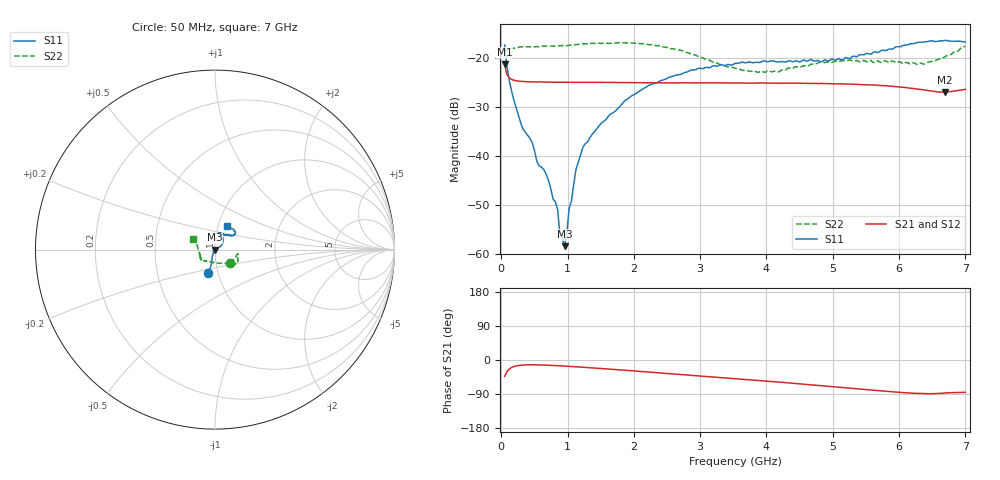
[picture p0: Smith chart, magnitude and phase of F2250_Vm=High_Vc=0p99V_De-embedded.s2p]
! Integrated Device Technology
! Corporate Headquarters
! 6024 Silver Creek Valley Road
! San Jose, CA 95138  USA
! Phone:  1-408-284-8200
! Toll Free:  1-800-223-1366
! Webpage:  http://www.idt.com/
! Timing and RF Division
! 515 Groton Road, Suite 102
! Westford, MA 01886-6024
! Device:  F2250
! Description: Voltage Variable RF Attenuator
! Frequency:  50.0 -  6000.00 MHz
! Package:  3x3 mm Thin QFN Plastic Package: 16 pin
! Ports:  2 RF, 3 DC
!  Pin  1  = GND
!  Pin  2  = NC
!  Pin  3  = RF1  = Port 1
!  Pin  4  = NC
!  Pin  5  = GND
!  Pin  6  = GND
!  Pin  7  = GND
!  Pin  8  = GND
!  Pin  9  = NC
!  Pin 10  = RF2  = Port 2
!  Pin 11  = NC
!  Pin 12  = GND
!  Pin 13  = GND
!  Pin 14  = VCNTRL
!  Pin 15  = VDD
!  Pin 16  = VMODE
! Vcntrl:  0.990 Volts
! Vmode:  +3.300 Volts
! Vdd:  +3.30  Volts
! Current:  1.325 mA
! Data:  The device was measured on a the F2250 evaluation board which has
!  individual transmission lines to the RF pins.  Data was collected
!  using a calibrated network analyzer.  The evaluation board was
!  de-embedded using a TRL calibration technique.
!  The reference plane is the edge of the package pin.
! Misc:  SN 10
!  Action Tracker AT0258
! Date Measured:  2014-11-26
! Date:  2015-10-15  MJV
! Note:
!  Integrated Device Technology supplies this data as a sample of measured
!  data at the package pin for this product.  Your particular data for this
!  product may vary.
!  Data was taken at 25 degrees C.
!  Integrated Device Technology reserves the right to change this data at anytime.
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# GHz S dB R 50
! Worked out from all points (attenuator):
!   201 points, 50 MHz to 7 GHz, reference 50 ohm
!   highest |S21| = -21.20 dB at 50 MHz (marker M1); lowest = -26.9 dB at 6.687 GHz (marker M2)
!   lowest |S11| = -58.4 dB at 953.5 MHz (marker M3), VSWR 1.00, Z = 49.9 - j0.0804 ohm
!   |S11| at or under -10 dB: start of sweep to end of sweep
!   |S22| runs from -22.9 to -16.8 dB; largest |S21 - S12| = 0.00023
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0.05  -17.25 -105.8  -21.20 -43.3  -21.21 -43.3  -19.21 -42.3
0.1195  -24.43 -106.8  -23.97 -24.0  -23.95 -24.0  -18.09 -15.0
0.189  -28.48 -112.3  -24.44 -17.4  -24.43 -17.3  -17.89 -11.6
0.328  -34.45 -120.6  -24.70 -13.3  -24.69 -13.3  -17.59 -10.6
0.467  -37.21 -130.2  -24.79 -12.7  -24.80 -12.7  -17.65 -11.8
0.5365  -41.02 -133.3  -24.81 -12.8  -24.79 -12.8  -17.57 -13.2
0.71025  -44.83 -142.4  -24.84 -13.9  -24.85 -13.9  -17.47 -16.2
0.84925  -50.87 -176.6  -24.86 -15.1  -24.86 -15.1  -17.43 -19.1
0.884  -55.84 175.0  -24.88 -15.4  -24.89 -15.4  -17.39 -20.0
0.9535  -58.38 -138.1  -24.88 -16.0  -24.87 -16.1  -17.43 -20.9
0.98825  -55.79 -31.7  -24.87 -16.4  -24.88 -16.4  -17.38 -21.4
1.023  -50.69 -1.0  -24.87 -16.7  -24.89 -16.7  -17.30 -21.6
1.12725  -42.64 14.3  -24.88 -17.8  -24.88 -17.8  -17.16 -23.3
1.2315  -38.14 17.5  -24.87 -19.1  -24.88 -19.1  -17.00 -25.2
1.857  -28.72 31.2  -24.91 -27.0  -24.93 -27.0  -16.79 -31.6
2.37825  -24.72 41.4  -24.96 -33.7  -24.97 -33.7  -17.35 -36.7
3.525  -21.00 69.3  -25.02 -49.1  -25.03 -49.2  -22.01 -74.3
4.18525  -20.70 75.9  -25.06 -58.2  -25.07 -58.3  -22.73 -115.0
4.7065  -20.49 70.7  -25.09 -66.0  -25.10 -66.0  -21.18 -134.3
5.85325  -18.05 39.3  -25.65 -83.2  -25.66 -83.4  -20.87 -153.2
6.68725  -16.32 47.0  -26.90 -87.2  -26.91 -87.3  -19.72 165.2
7  -16.62 61.9  -26.31 -85.3  -26.30 -85.4  -17.48 155.0
